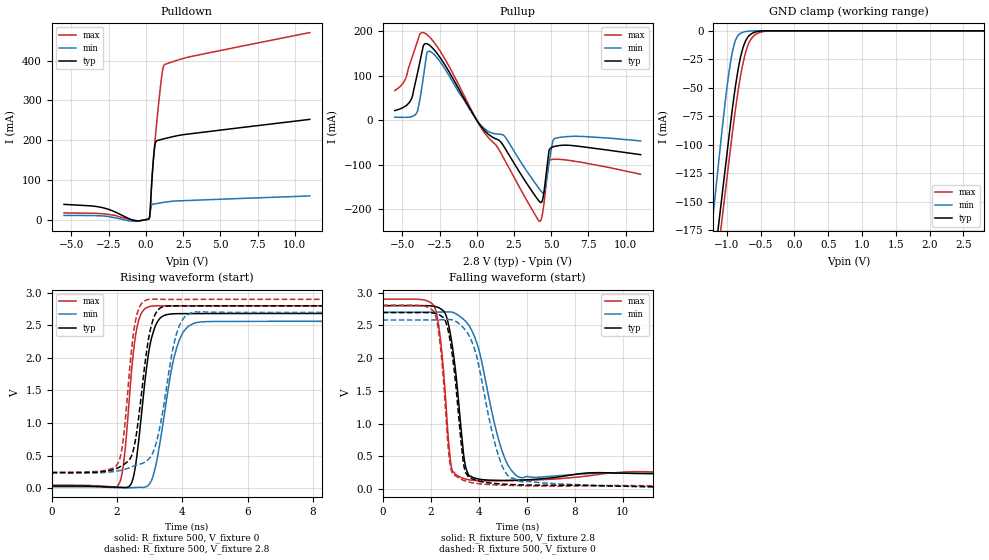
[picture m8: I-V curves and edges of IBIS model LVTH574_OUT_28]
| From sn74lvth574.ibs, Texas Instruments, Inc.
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[Model]   LVTH574_OUT_28
Model_type  3-state
Enable   Active-Low
Vref =   0
Rref =   500
Cref =   50p
Vmeas =   1.5
| variable   typ   min   max
C_comp   5.78pF   4.76pF   7.95pF
| C_pullup   4.82pF   0.33pF   7.52pF
| C_pulldown   6.03pF   1.99pF   10.06pF
| C_tri-state   5.78pF   4.76pF   7.95pF
[Temperature Range]   40   -40   100
| Ambient temperature   25   -40   85
[Voltage range]   2.8   2.7   2.9
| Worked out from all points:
|   slope of the pulldown table from 0 to 0.42 V, typ, clamps not added: 3.84 ohm
|   slope of the pullup table from 0 to 0.42 V, typ, clamps not added: 21.9 ohm
|   GND clamp passes 1 mA (typ) near -0.58 V on its own axis
|   rising waveform, R_fixture 500, V_fixture 0: 20-80 % time 369ps typ, 515ps min, 293ps max; typ from 0.032 V to 2.68 V
|   falling waveform, R_fixture 500, V_fixture 2.8: 20-80 % time 454ps typ, 911ps min, 354ps max; typ from 2.8 V to 0.238 V
|   rising waveform, R_fixture 500, V_fixture 2.8: 20-80 % time 396ps typ, 523ps min, 305ps max; typ from 0.238 V to 2.8 V
|   falling waveform, R_fixture 500, V_fixture 0: 20-80 % time 457ps typ, 920ps min, 358ps max; typ from 2.69 V to 0.032 V
[GND Clamp]
| LVTH574_OUT_28
|   Voltage   I(typ)   I(min)   I(max)
-5.5V     -2.851A    -3.021A    -2.852A
-1.22V    -219.7mA   -171mA     -239.9mA
-1.18V    -199.4mA   -148.2mA   -219.5mA
-1.075V   -146.2mA   -88.9mA    -166.9mA
-975mV    -95.92mA   -38.87mA   -117.3mA
-925mV    -71.24mA   -20.27mA   -92.6mA
-875mV    -49.22mA   -8.568mA   -69.52mA
-800mV    -23.53mA   -2.203mA   -40.17mA
-725mV    -8.992mA   -701.6uA   -19.44mA
-650mV    -3.105mA   -178.1uA   -7.929mA
-575mV    -985.7uA   -11.41uA   -3.152mA
2.8V      28.2pA     20.95pA    1.193nA
[Pulldown]
| LVTH574_OUT_28
|   Voltage   I(typ)   I(min)   I(max)
-5.5V     38.16mA    10.26mA    16.67mA
-2.92V    29.95mA    9.053mA    14.61mA
-680mV    -3.137mA   -4.471mA   -2.335mA
215mV     2.328mA    2.784mA    2.242mA
285mV     22.67mA    17.64mA    18.47mA
365mV     76.4mA     34.67mA    76.09mA
465mV     132.9mA    38.47mA    134.9mA
620mV     189.6mA    39.58mA    203.1mA
1.05V     201.9mA    42.37mA    358.1mA
1.155V    202.9mA    43.01mA    382.5mA
1.26V     203.9mA    43.62mA    390.4mA
11V       252.3mA    59.42mA    471mA
[Pullup]
| LVTH574_OUT_28
|   Voltage   I(typ)   I(min)   I(max)
-5.5V     21.77mA    6.604mA    66.92mA
-4.47V    42.68mA    7.356mA    128.3mA
-4.02V    99.38mA    17.02mA    173.5mA
-3.585V   167.5mA    96.63mA    196.9mA
-3.23V    169.9mA    155mA      189.1mA
1.9V      -63.21mA   -37.14mA   -90.92mA
4.215V    -183mA     -154.8mA   -227.1mA
4.55V     -151.6mA   -160.2mA   -176.4mA
4.815V    -77.28mA   -105.1mA   -97.38mA
4.96V     -62.75mA   -73.72mA   -89.02mA
5.58V     -56.76mA   -38.47mA   -87.96mA
11V       -77.42mA   -46.53mA   -121.5mA
[Ramp]
| LVTH574_OUT_28
| variable   typ   min   max
dV/dt_r   1.61/3.83E-10   1.54/5.21E-10   1.67/2.97E-10
dV/dt_f   1.60/4.70E-10   1.51/9.44E-10   1.66/3.77E-10
R_load = 500
[Rising Waveform]
| LVTH574_OUT_28
R_fixture =   500
C_fixture =   0
L_fixture =   0
V_fixture =   0
V_fixture_min = 0
V_fixture_max = 0
|   Time   V(typ)   V(min)   V(max)
0s        32.2mV     19.9mV     45.21mV
2.05ns    13.36mV    5.095mV    55.25mV
2.215ns   9.907mV    3.695mV    436.6mV
2.44ns    72.25mV    5.597mV    1.77V
2.595ns   442mV      10.15mV    2.424V
3.05ns    2.29V      111.8mV    2.796V
3.325ns   2.614V     725.4mV    2.8V
3.84ns    2.679V     2.175V     2.799V
4.58ns    2.681V     2.553V     2.8V
50ns      2.684V     2.563V     2.801V
[Falling Waveform]
| LVTH574_OUT_28
R_fixture =   500
C_fixture =   0
L_fixture =   0
V_fixture =   2.8
V_fixture_min = 2.7
V_fixture_max = 2.9
|   Time   V(typ)   V(min)   V(max)
0s        2.8V       2.7V       2.9V
2.125ns   2.792V     2.701V     2.811V
2.365ns   2.765V     2.702V     2.429V
2.61ns    2.681V     2.705V     1.466V
2.895ns   2.212V     2.701V     296.7mV
3.38ns    517.6mV    2.589V     163.4mV
3.62ns    201.1mV    2.485V     142.6mV
4.975ns   134.1mV    585.8mV    127.6mV
5.77ns    139.5mV    175.1mV    133mV
50ns      237.6mV    231.9mV    243.7mV
[Rising Waveform]
| LVTH574_OUT_28
R_fixture =   500
C_fixture =   0
L_fixture =   0
V_fixture =   2.8
V_fixture_min = 2.7
V_fixture_max = 2.9
|   Time   V(typ)   V(min)   V(max)
0s        238mV      232.1mV    244.1mV
2.02ns    308.9mV    263.5mV    375.1mV
2.19ns    356.5mV    282.4mV    745.2mV
2.44ns    489.3mV    324.8mV    2.106V
2.56ns    726.8mV    349.4mV    2.551V
2.97ns    2.305V     445mV      2.899V
3.26ns    2.737V     814.4mV    2.9V
3.84ns    2.799V     2.398V     2.898V
4.38ns    2.798V     2.707V     2.899V
50ns      2.8V       2.7V       2.9V
[Falling Waveform]
| LVTH574_OUT_28
R_fixture =   500
C_fixture =   0
L_fixture =   0
V_fixture =   0
V_fixture_min = 0
V_fixture_max = 0
|   Time   V(typ)   V(min)   V(max)
0s        2.695V     2.582V     2.808V
2.125ns   2.687V     2.583V     2.718V
2.355ns   2.662V     2.584V     2.351V
2.59ns    2.587V     2.587V     1.413V
2.88ns    2.111V     2.587V     269.4mV
3.38ns    372.3mV    2.458V     134.4mV
3.82ns    145.5mV    2.152V     91.95mV
4.9ns     80.88mV    431.2mV    62.47mV
5.805ns   64.89mV    113.1mV    52.86mV
50ns      32.22mV    19.91mV    45.26mV
